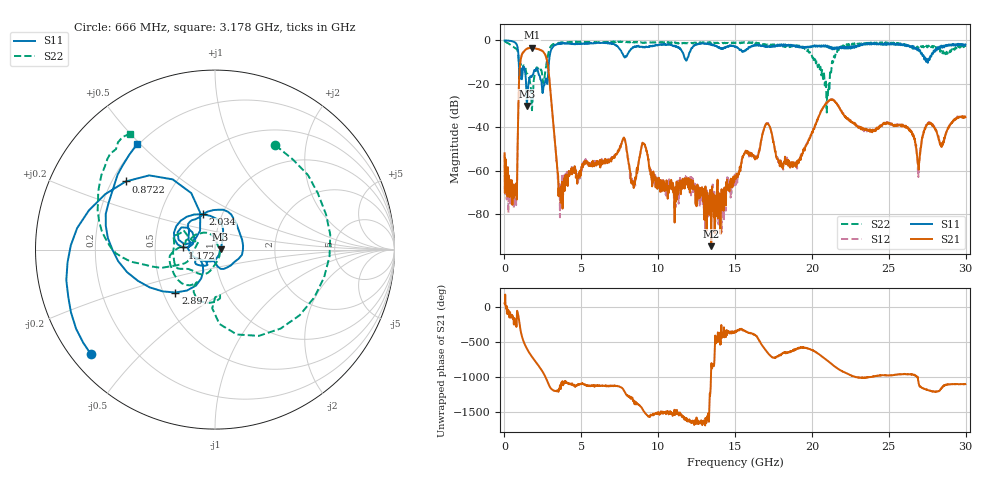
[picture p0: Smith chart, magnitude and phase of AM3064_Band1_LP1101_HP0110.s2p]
# Hz S DB R 50.0
!freq dBS11 angS11 dBS21 angS21 dBS12 angS12 dBS22 angS22
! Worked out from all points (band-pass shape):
!   1600 points, 10 MHz to 29.98 GHz, reference 50 ohm
!   highest |S21| = -3.41 dB at 1.791 GHz (marker M1); lowest = -94.6 dB at 13.45 GHz (marker M2)
!   |S21| within 3 dB of the highest: 1.142 GHz to 2.635 GHz (1.493 GHz wide, 79.1 % of centre)
!   lowest |S11| = -30.1 dB at 1.453 GHz (marker M3), VSWR 1.06, Z = 53.2 + j0.2 ohm
!   |S11| at or under -10 dB: 931.8 MHz to 2.893 GHz (1.962 GHz wide, 103 % of centre); 27.52394 GHz to 27.55045 GHz (26.5 MHz wide, 0.0962 % of centre)
!   |S22| runs from -33.2 to -0.4 dB; largest |S21 - S12| = 0.009
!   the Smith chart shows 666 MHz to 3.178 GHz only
!   S11 on the Smith chart (normalised r, x): 666 MHz: 0.06, -0.36; 872.2 MHz: 0.26, +0.32; 1.172 GHz: 0.69, +0.02; 2.034 GHz: 0.81, +0.33; 2.897 GHz: 0.58, -0.31; 3.178 GHz: 0.19, +0.49
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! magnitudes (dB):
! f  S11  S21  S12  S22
! 10 MHz  -0.1  -51.9  -52.4  -0.4
! 666 MHz  -0.9  -66.5  -67.3  -3.5
! 872.2 MHz  -4.1  -42.1  -42.0  -5.4
! 1.172 GHz  -14.9  -5.9  -5.9  -13.0
! 1.453 GHz  -30.1  -3.9  -3.8  -15.5
! 1.791 GHz  -16.4  -3.4  -3.4  -32.1
! 2.034 GHz  -13.6  -3.7  -3.7  -13.9
! 2.897 GHz  -9.8  -16.1  -16.0  -4.7
! 3.178 GHz  -2.7  -38.6  -38.6  -1.9
! 3.665 GHz  -1.6  -74.6  -66.6  -1.0
! 5.015 GHz  -1.6  -58.0  -59.4  -0.6
! 7.751 GHz  -7.2  -45.0  -45.0  -0.7
! 10 GHz  -2.1  -66.2  -64.6  -0.9
! 13.45 GHz  -1.8  -94.6  -70.6  -1.1
! 15 GHz  -2.8  -63.6  -63.0  -1.3
! 17.05 GHz  -2.9  -38.4  -38.1  -2.2
! 18.04 GHz  -2.0  -57.9  -57.3  -2.2
! 19.99 GHz  -3.1  -42.7  -42.7  -6.9
! 20.98 GHz  -2.5  -28.6  -28.3  -26.1
! 25 GHz  -1.3  -38.1  -38.1  -1.2
! 26.94 GHz  -4.4  -59.4  -56.1  -3.3
! 29.98 GHz  -1.9  -35.3  -35.3  -3.0
